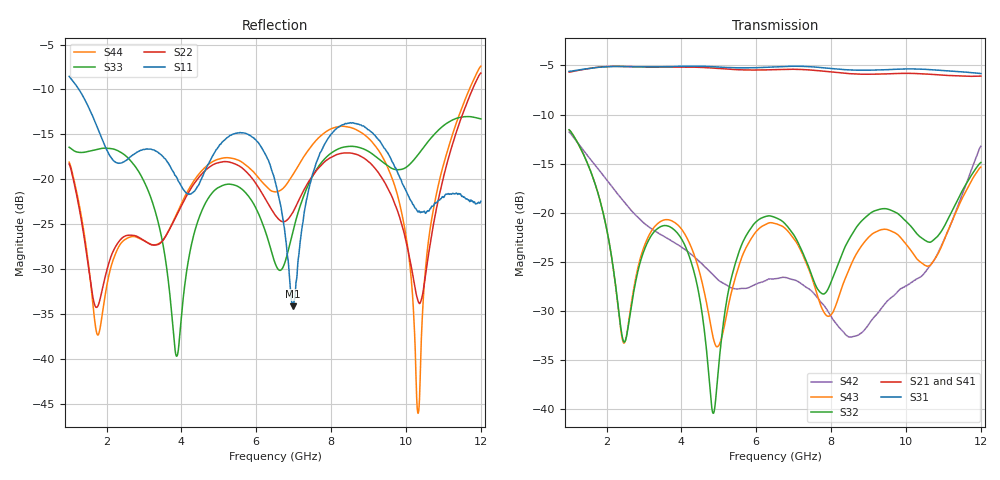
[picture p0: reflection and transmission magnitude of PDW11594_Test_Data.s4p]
!Keysight Technologies,N5227B,US57180409,A.15.40.08
!Date: Saturday, April 20, 2024 08:37:13
!Correction: S11(C  4-Port  )
!S12(C  4-Port  )
!S13(C  4-Port  )
!S14(C  4-Port  )
!S21(C  4-Port  )
!S22(C  4-Port  )
!S23(C  4-Port  )
!S24(C  4-Port  )
!S31(C  4-Port  )
!S32(C  4-Port  )
!S33(C  4-Port  )
!S34(C  4-Port  )
!S41(C  4-Port  )
!S42(C  4-Port  )
!S43(C  4-Port  )
!S44(C  4-Port  )
!S4P File: Measurements: <S11,S12,S13,S14>,
!<S21,S22,S23,S24>,
!<S31,S32,S33,S34>,
!<S41,S42,S43,S44>:
# Hz S  dB  R 50
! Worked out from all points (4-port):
!   3201 points, 1 GHz to 12 GHz, reference 50 ohm
!   strongest paths, dB at 1 GHz, 3.75 GHz, 6.5 GHz, 9.25 GHz, 12 GHz:
!     S31: -5.6, -5.1, -5.1, -5.5, -5.8
!     S21: -5.7, -5.2, -5.4, -5.9, -6.1
!     S41: -5.7, -5.2, -5.5, -6.0, -6.6
!     S32: -11.6, -21.6, -20.5, -19.7, -14.9
!     S43: -11.6, -20.8, -21.1, -21.9, -15.3
!     S42: -11.8, -22.9, -26.7, -30.2, -13.2
!   lowest |S11| = -34.2 dB at 6.985 GHz (marker M1), VSWR 1.04, Z = 49.3 + j1.8 ohm
!   |S11| at or under -10 dB: 1.261 GHz to end of sweep
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1e9  -8.54 132.1  -5.67 -64.4  -5.60 -65.3  -5.70 -64.7
     -5.68 -64.5  -18.30 32.0  -11.55 -72.1  -11.79 -118.3
     -5.60 -65.3  -11.56 -72.1  -16.44 116.6  -11.57 -72.2
     -5.71 -64.7  -11.79 -118.3  -11.57 -72.3  -18.10 32.6
3.87375e9  -19.80 119.3  -5.16 96.2  -5.10 96.0  -5.20 94.9
           -5.16 96.1  -24.02 117.4  -21.99 -96.5  -23.19 -91.7
           -5.10 96.0  -21.99 -96.4  -39.72 -112.2  -21.14 -90.4
           -5.21 94.9  -23.18 -91.7  -21.14 -90.5  -23.89 110.0
4.85e9  -17.31 150.9  -5.26 27.4  -5.12 27.2  -5.32 25.9
        -5.27 27.3  -18.37 78.9  -40.45 114.8  -26.33 141.9
        -5.12 27.1  -40.44 114.8  -21.39 98.1  -32.77 -105.5
        -5.33 25.8  -26.33 141.9  -32.77 -105.4  -18.00 74.7
6.984688e9  -34.16 110.9  -5.39 -122.6  -5.09 -122.9  -5.46 -124.8
            -5.39 -122.5  -23.63 52.0  -22.17 -93.6  -26.82 -141.6
            -5.08 -123.0  -22.16 -93.7  -25.71 84.9  -22.54 -148.3
            -5.46 -124.8  -26.82 -141.6  -22.55 -148.1  -19.45 52.0
9.380625e9  -16.25 0.9  -5.87 64.7  -5.45 63.7  -6.01 62.3
            -5.87 64.8  -20.01 -32.4  -19.59 -102.5  -29.55 -124.2
            -5.44 63.7  -19.59 -102.6  -18.10 -0.9  -21.71 -82.0
            -6.00 62.3  -29.54 -124.3  -21.70 -81.9  -17.58 -36.6
1.03225e10  -23.66 -139.5  -5.83 -6.0  -5.35 -7.6  -5.91 -8.9
            -5.83 -6.0  -33.56 -133.1  -22.26 -129.1  -26.68 106.4
            -5.36 -7.5  -22.27 -129.1  -17.26 8.9  -24.84 -116.3
            -5.91 -9.0  -26.68 106.3  -24.83 -116.4  -46.08 -163.0
1.2e10  -22.45 51.7  -6.07 -134.4  -5.79 -139.1  -6.55 -137.6
        -6.08 -134.3  -8.17 51.1  -14.87 -147.3  -13.22 -128.5
        -5.82 -139.1  -14.88 -147.4  -13.28 -30.5  -15.36 -145.8
        -6.57 -137.7  -13.22 -128.7  -15.35 -146.0  -7.41 45.2
